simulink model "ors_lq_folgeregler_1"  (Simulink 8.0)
settings: Solver=ode45  SolverMode=SingleTasking  StartTime=0.0  StopTime=10  FixedStep=0.01  MaxStep=0.01  RelTol=1e-3  AbsTol=1e-3
undefined symbols (not defined in the file or in its folder): k

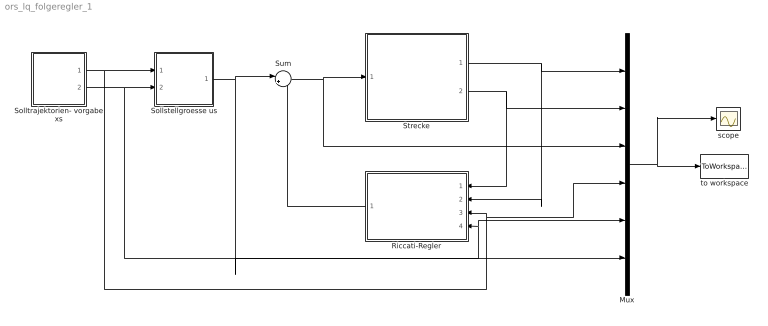
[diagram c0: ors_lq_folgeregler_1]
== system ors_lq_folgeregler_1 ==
  Mux : Mux  Inputs=6
  Riccati-Regler : Subsystem
  Sollstellgroesse us : Subsystem
  Solltrajektorien- vorgabe xs : Subsystem
  Strecke : Subsystem
  Sum : Sum  Inputs=|+-
  scope : Scope
  to workspace : ToWorkspace  VariableName=simout  SampleTime=-1  SaveFormat=Structure With Time
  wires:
  Strecke/1(x1) -> Riccati-Regler/2(x1), Mux/1
  Strecke/2(x2) -> Riccati-Regler/1(x2), Mux/2
  Mux/1 -> to workspace/1, scope/1
  Solltrajektorien- vorgabe xs/1(x1s) -> Sollstellgroesse us/1(x1s), Riccati-Regler/3(x1s), Mux/4
  Solltrajektorien- vorgabe xs/2(x2s) -> Sollstellgroesse us/2(x2s), Riccati-Regler/4(x2s), Mux/5
  Sollstellgroesse us/1(us) -> Sum/1, Mux/6
  Sum/1 -> Strecke/1(u), Mux/3
  Riccati-Regler/1(-du) -> Sum/2

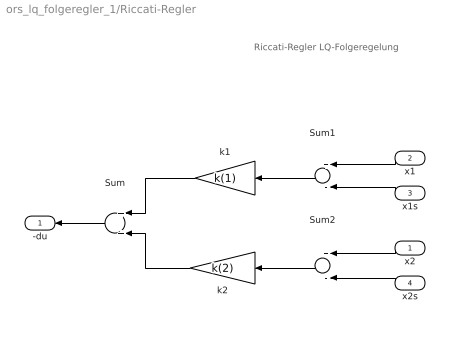
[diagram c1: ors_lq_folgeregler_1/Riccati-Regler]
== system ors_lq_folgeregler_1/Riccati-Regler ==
  note: Riccati-Regler LQ-Folgeregelung
  x2 : Inport
  x1 : Inport  Port=2
  x1s : Inport  Port=3
  x2s : Inport  Port=4
  Sum : Sum
  Sum1 : Sum  Inputs=+-
  Sum2 : Sum  Inputs=+-
  k1 : Gain  Gain=k(1)
  k2 : Gain  Gain=k(2)
  -du : Outport  InitialOutput=0
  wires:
  Sum1/1 -> k1/1
  Sum2/1 -> k2/1
  x2/1 -> Sum2/1
  Sum/1 -> -du/1
  k2/1 -> Sum/2
  k1/1 -> Sum/1
  x1/1 -> Sum1/1
  x1s/1 -> Sum1/2
  x2s/1 -> Sum2/2

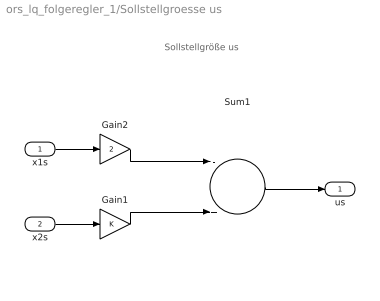
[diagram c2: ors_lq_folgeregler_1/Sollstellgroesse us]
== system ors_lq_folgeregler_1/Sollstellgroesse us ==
  note: Sollstellgröße us
  x1s : Inport
  x2s : Inport  Port=2
  Gain1 : Gain
  Gain2 : Gain  Gain=2
  Sum1 : Sum  Inputs=-+
  us : Outport  InitialOutput=0
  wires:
  Gain2/1 -> Sum1/1
  Gain1/1 -> Sum1/2
  Sum1/1 -> us/1
  x1s/1 -> Gain2/1
  x2s/1 -> Gain1/1

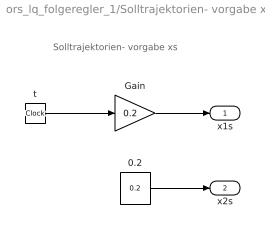
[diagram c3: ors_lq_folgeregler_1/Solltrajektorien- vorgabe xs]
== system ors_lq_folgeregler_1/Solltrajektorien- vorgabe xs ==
  note: Solltrajektorien- vorgabe xs
  0.2 : Constant  Value=0.2
  Gain : Gain  Gain=0.2
  t : Clock
  x1s : Outport  InitialOutput=0
  x2s : Outport  Port=2  InitialOutput=0
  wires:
  0.2/1 -> x2s/1
  t/1 -> Gain/1
  Gain/1 -> x1s/1

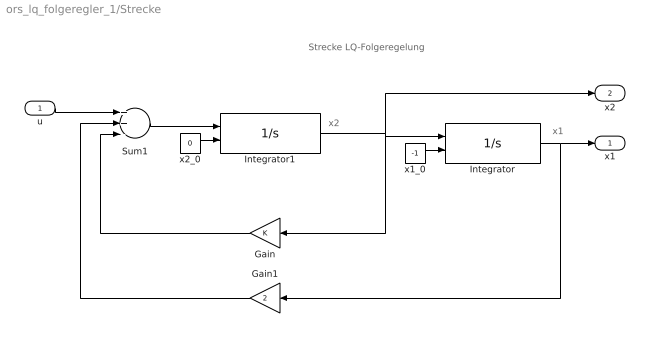
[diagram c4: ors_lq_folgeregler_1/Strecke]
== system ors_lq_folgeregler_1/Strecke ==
  note: x1
  note: x2
  note: Strecke LQ-Folgeregelung
  u : Inport
  Gain : Gain
  Gain1 : Gain  Gain=2
  Integrator : Integrator  InitialConditionSource=external
  Integrator1 : Integrator  InitialConditionSource=external
  Sum1 : Sum  Inputs=++-
  x1_0 : Constant  Value=-1
  x2_0 : Constant  Value=0
  x1 : Outport  InitialOutput=0
  x2 : Outport  Port=2  InitialOutput=0
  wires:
  Integrator1/1 -> Integrator/1, Gain/1, x2/1
  Sum1/1 -> Integrator1/1
  Gain/1 -> Sum1/3
  Gain1/1 -> Sum1/2
  u/1 -> Sum1/1
  Integrator/1 -> Gain1/1, x1/1
  x2_0/1 -> Integrator1/2
  x1_0/1 -> Integrator/2
